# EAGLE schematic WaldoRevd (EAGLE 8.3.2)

## Sheet 1 of 6: Microcontroller Module
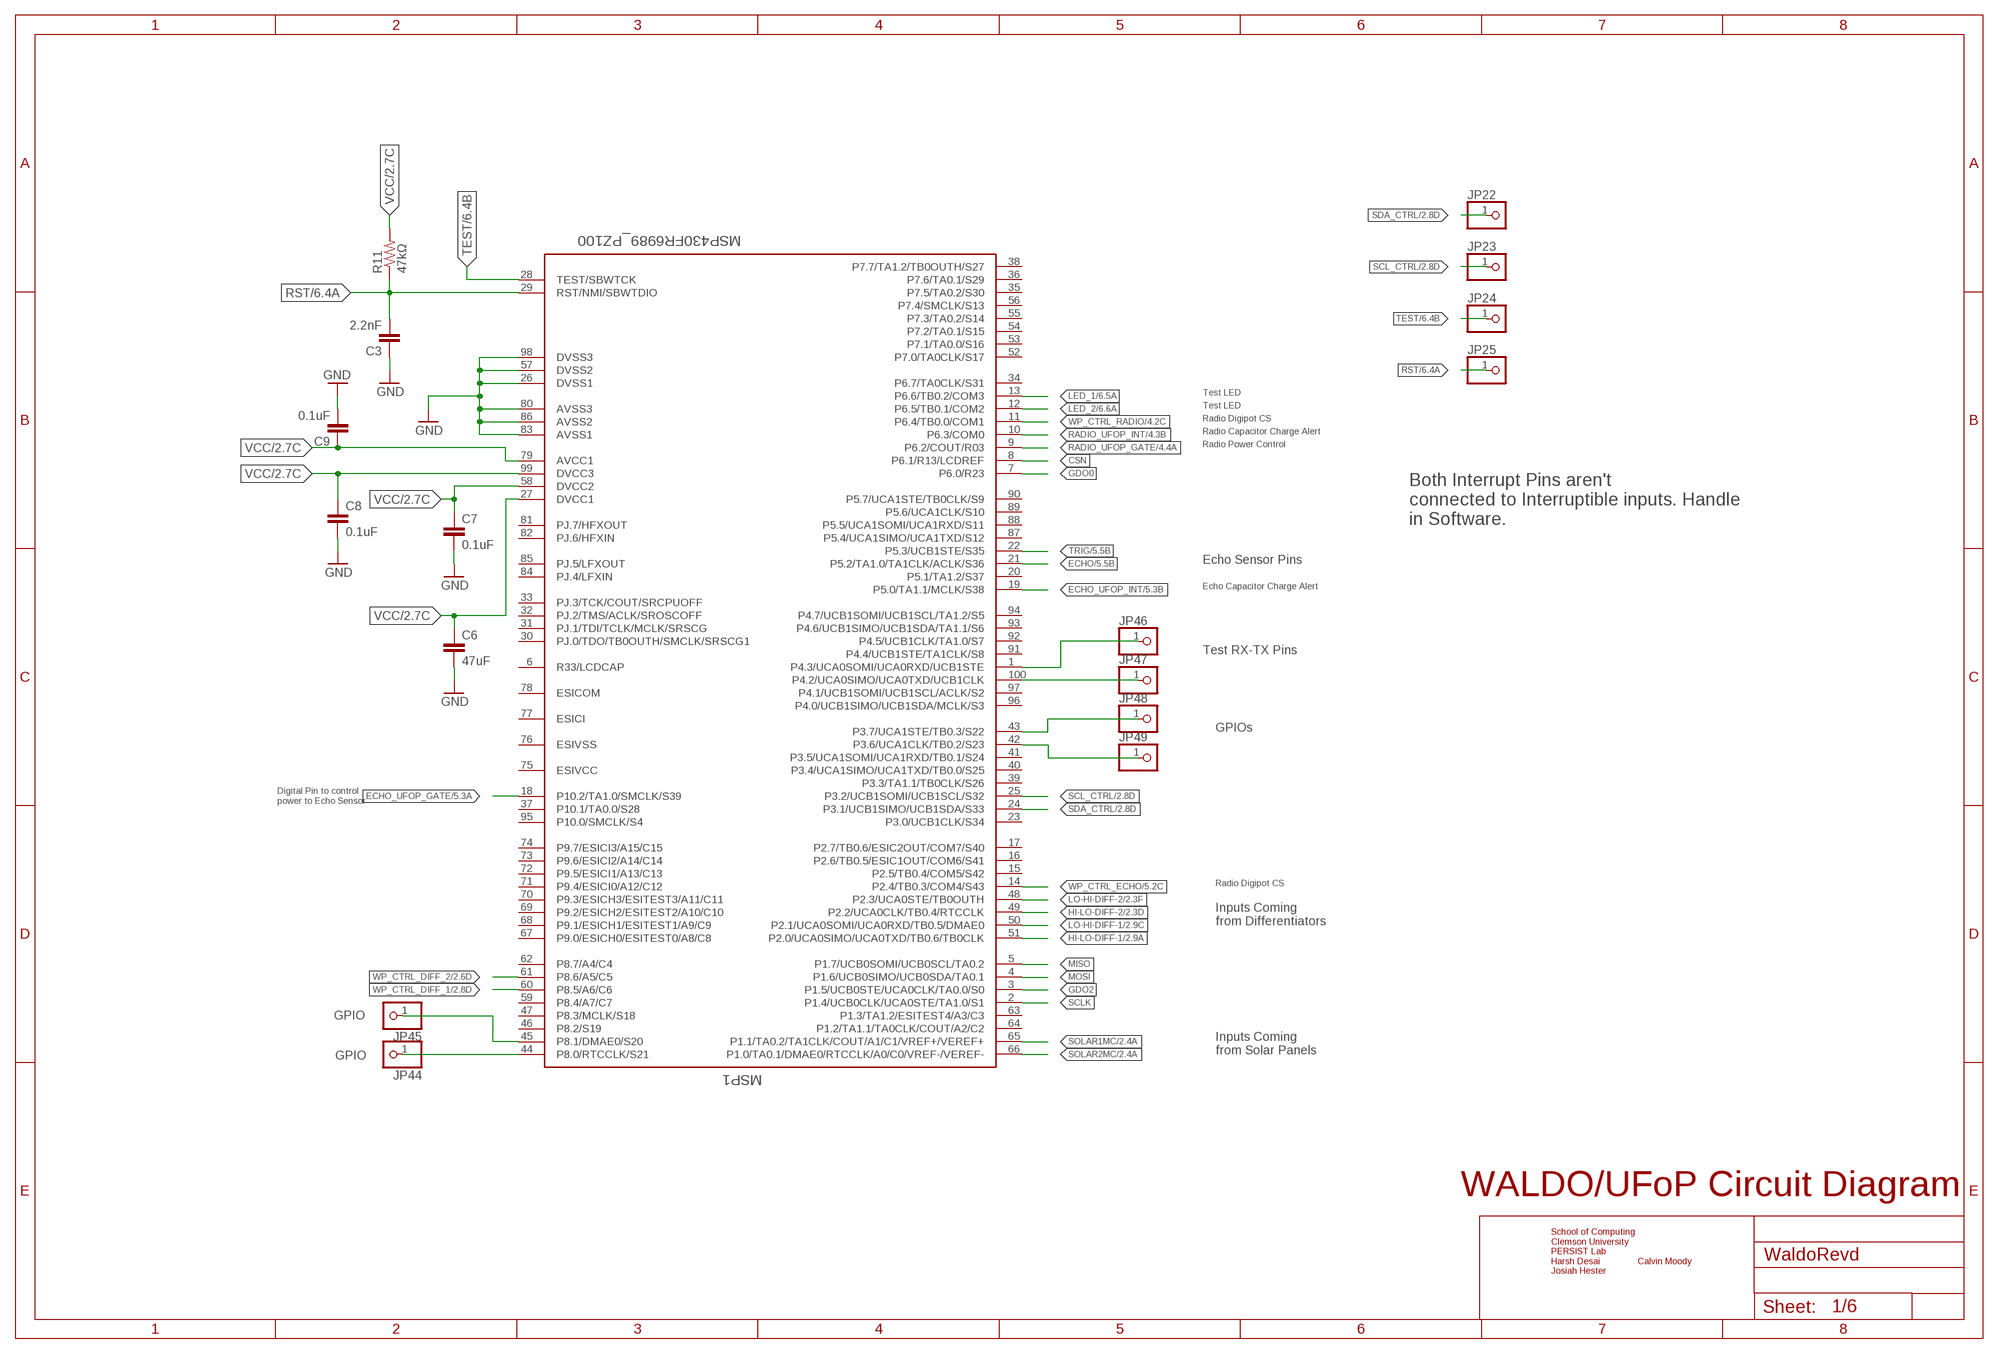
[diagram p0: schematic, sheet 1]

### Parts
C3  2.2nF  CAP0805  [0805]
C6  47uF  CAP0805  [0805]
C7  0.1uF  CAP0805  [0805]
C8  0.1uF  CAP0805  [0805]
C9  0.1uF  CAP0805  [0805]
JP22  PINHD-1X1  [1X01]
JP23  PINHD-1X1  [1X01]
JP24  PINHD-1X1  [1X01]
JP25  PINHD-1X1  [1X01]
JP44  PINHD-1X1  [1X01]
JP45  PINHD-1X1  [1X01]
JP46  PINHD-1X1  [1X01]
JP47  PINHD-1X1  [1X01]
JP48  PINHD-1X1  [1X01]
JP49  PINHD-1X1  [1X01]
MSP1  MSP430FR6989_PZ100  [PZ100]
R11  47kΩ  RESISTOR0805-RES  [0805]

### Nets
CSN: MSP1.8(P6.1/R13/LCDREF) ; also sheet 4
ECHO: MSP1.21(P5.2/TA1.0/TA1CLK/ACLK/S36) ; also sheet 5
ECHO_UFOP_GATE: MSP1.18(P10.2/TA1.0/SMCLK/S39) ; also sheet 5
ECHO_UFOP_INT: MSP1.19(P5.0/TA1.1/MCLK/S38) ; also sheet 5
GDO0: MSP1.7(P6.0/R23) ; also sheet 4
GDO2: MSP1.3(P1.5/UCB0STE/UCA0CLK/TA0.0/S0) ; also sheet 4
GND: C3.1 C6.2 C7.2 C8.2 C9.2 MSP1.26(DVSS1) MSP1.57(DVSS2) MSP1.80(AVSS3) MSP1.83(AVSS1) MSP1.86(AVSS2) MSP1.98(DVSS3) ; also sheet 2,3,4,5,6
HI-LO-DIFF-1: MSP1.51(P2.0/UCA0SIMO/UCA0TXD/TB0.6/TB0CLK) ; also sheet 2
HI-LO-DIFF-2: MSP1.49(P2.2/UCA0CLK/TB0.4/RTCCLK) ; also sheet 2
LED_1: MSP1.13(P6.6/TB0.2/COM3) ; also sheet 6
LED_2: MSP1.12(P6.5/TB0.1/COM2) ; also sheet 6
LO-HI-DIFF-1: MSP1.50(P2.1/UCA0SOMI/UCA0RXD/TB0.5/DMAE0) ; also sheet 2
LO-HI-DIFF-2: MSP1.48(P2.3/UCA0STE/TB0OUTH) ; also sheet 2
MISO: MSP1.5(P1.7/UCB0SOMI/UCB0SCL/TA0.2) ; also sheet 4
MOSI: MSP1.4(P1.6/UCB0SIMO/UCB0SDA/TA0.1) ; also sheet 4
N$1: JP44.1 MSP1.44(P8.0/RTCCLK/S21)
N$2: JP45.1 MSP1.45(P8.1/DMAE0/S20)
N$3: JP46.1 MSP1.1(P4.3/UCA0SOMI/UCA0RXD/UCB1STE)
N$5: JP47.1 MSP1.100(P4.2/UCA0SIMO/UCA0TXD/UCB1CLK)
N$6: JP49.1 MSP1.42(P3.6/UCA1CLK/TB0.2/S23)
N$10: JP48.1 MSP1.43(P3.7/UCA1STE/TB0.3/S22)
RADIO_UFOP_GATE: MSP1.9(P6.2/COUT/R03) ; also sheet 4
RADIO_UFOP_INT: MSP1.10(P6.3/COM0) ; also sheet 4
RST: C3.2 JP25.1 MSP1.29(RST/NMI/SBWTDIO) R11.1 ; also sheet 6
SCL_CTRL: JP23.1 MSP1.25(P3.2/UCB1SOMI/UCB1SCL/S32) ; also sheet 2,4,5,6
SCLK: MSP1.2(P1.4/UCB0CLK/UCA0STE/TA1.0/S1) ; also sheet 4
SDA_CTRL: JP22.1 MSP1.24(P3.1/UCB1SIMO/UCB1SDA/S33) ; also sheet 2,4,5,6
SOLAR1MC: MSP1.65(P1.1/TA0.2/TA1CLK/COUT/A1/C1/VREF+/VEREF+) ; also sheet 2
SOLAR2MC: MSP1.66(P1.0/TA0.1/DMAE0/RTCCLK/A0/C0/VREF-/VEREF-) ; also sheet 2
TEST: JP24.1 MSP1.28(TEST/SBWTCK) ; also sheet 6
TRIG: MSP1.22(P5.3/UCB1STE/S35) ; also sheet 5
VCC: C6.1 C7.1 C8.1 C9.1 MSP1.27(DVCC1) MSP1.58(DVCC2) MSP1.79(AVCC1) MSP1.99(DVCC3) R11.2 ; also sheet 2,3,6
WP_CTRL_DIFF_1: MSP1.60(P8.5/A6/C6) ; also sheet 2
WP_CTRL_DIFF_2: MSP1.61(P8.6/A5/C5) ; also sheet 2
WP_CTRL_ECHO: MSP1.14(P2.4/TB0.3/COM4/S43) ; also sheet 5
WP_CTRL_RADIO: MSP1.11(P6.4/TB0.0/COM1) ; also sheet 4
Unconnected: MSP1.6(R33/LCDCAP) MSP1.15(P2.5/TB0.4/COM5/S42) MSP1.16(P2.6/TB0.5/ESIC1OUT/COM6/S41) MSP1.17(P2.7/TB0.6/ESIC2OUT/COM7/S40) MSP1.20(P5.1/TA1.2/S37) MSP1.23(P3.0/UCB1CLK/S34) MSP1.30(PJ.0/TDO/TB0OUTH/SMCLK/SRSCG1) MSP1.31(PJ.1/TDI/TCLK/MCLK/SRSCG) MSP1.32(PJ.2/TMS/ACLK/SROSCOFF) MSP1.33(PJ.3/TCK/COUT/SRCPUOFF) MSP1.34(P6.7/TA0CLK/S31) MSP1.35(P7.5/TA0.2/S30) MSP1.36(P7.6/TA0.1/S29) MSP1.37(P10.1/TA0.0/S28) MSP1.38(P7.7/TA1.2/TB0OUTH/S27) MSP1.39(P3.3/TA1.1/TB0CLK/S26) MSP1.40(P3.4/UCA1SIMO/UCA1TXD/TB0.0/S25) MSP1.41(P3.5/UCA1SOMI/UCA1RXD/TB0.1/S24) MSP1.46(P8.2/S19) MSP1.47(P8.3/MCLK/S18) MSP1.52(P7.0/TA0CLK/S17) MSP1.53(P7.1/TA0.0/S16) MSP1.54(P7.2/TA0.1/S15) MSP1.55(P7.3/TA0.2/S14) MSP1.56(P7.4/SMCLK/S13) MSP1.59(P8.4/A7/C7) MSP1.62(P8.7/A4/C4) MSP1.63(P1.3/TA1.2/ESITEST4/A3/C3) MSP1.64(P1.2/TA1.1/TA0CLK/COUT/A2/C2) MSP1.67(P9.0/ESICH0/ESITEST0/A8/C8) MSP1.68(P9.1/ESICH1/ESITEST1/A9/C9) MSP1.69(P9.2/ESICH2/ESITEST2/A10/C10) MSP1.70(P9.3/ESICH3/ESITEST3/A11/C11) MSP1.71(P9.4/ESICI0/A12/C12) MSP1.72(P9.5/ESICI1/A13/C13) MSP1.73(P9.6/ESICI2/A14/C14) MSP1.74(P9.7/ESICI3/A15/C15) MSP1.75(ESIVCC) MSP1.76(ESIVSS) MSP1.77(ESICI) MSP1.78(ESICOM) MSP1.81(PJ.7/HFXOUT) MSP1.82(PJ.6/HFXIN) MSP1.84(PJ.4/LFXIN) MSP1.85(PJ.5/LFXOUT) MSP1.87(P5.4/UCA1SIMO/UCA1TXD/S12) MSP1.88(P5.5/UCA1SOMI/UCA1RXD/S11) MSP1.89(P5.6/UCA1CLK/S10) MSP1.90(P5.7/UCA1STE/TB0CLK/S9) MSP1.91(P4.4/UCB1STE/TA1CLK/S8) MSP1.92(P4.5/UCB1CLK/TA1.0/S7) MSP1.93(P4.6/UCB1SIMO/UCB1SDA/TA1.1/S6) MSP1.94(P4.7/UCB1SOMI/UCB1SCL/TA1.2/S5) MSP1.95(P10.0/SMCLK/S4) MSP1.96(P4.0/UCB1SIMO/UCB1SDA/MCLK/S3) MSP1.97(P4.1/UCB1SOMI/UCB1SCL/ACLK/S2)

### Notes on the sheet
- Test LED
- Test LED
- Radio Digipot CS
- Radio Capacitor Charge Alert
- Radio Power Control
- Both Interrupt Pins aren't 
  connected to Interruptible inputs. Handle
  in Software.
- Echo Sensor Pins
- Echo Capacitor Charge Alert
- Test RX-TX Pins
- GPIOs
- Digital Pin to control 
  power to Echo Sensor
- Radio Digipot CS
- Inputs Coming 
  from Differentiators
- GPIO
- Inputs Coming 
  from Solar Panels
- GPIO
- WALDO/UFoP Circuit Diagram
- School of Computing
  Clemson University
  PERSIST Lab
  Harsh Desai               Calvin Moody
  Josiah Hester

## Sheet 2 of 6: Solar Panels + Processing (Differentiators)
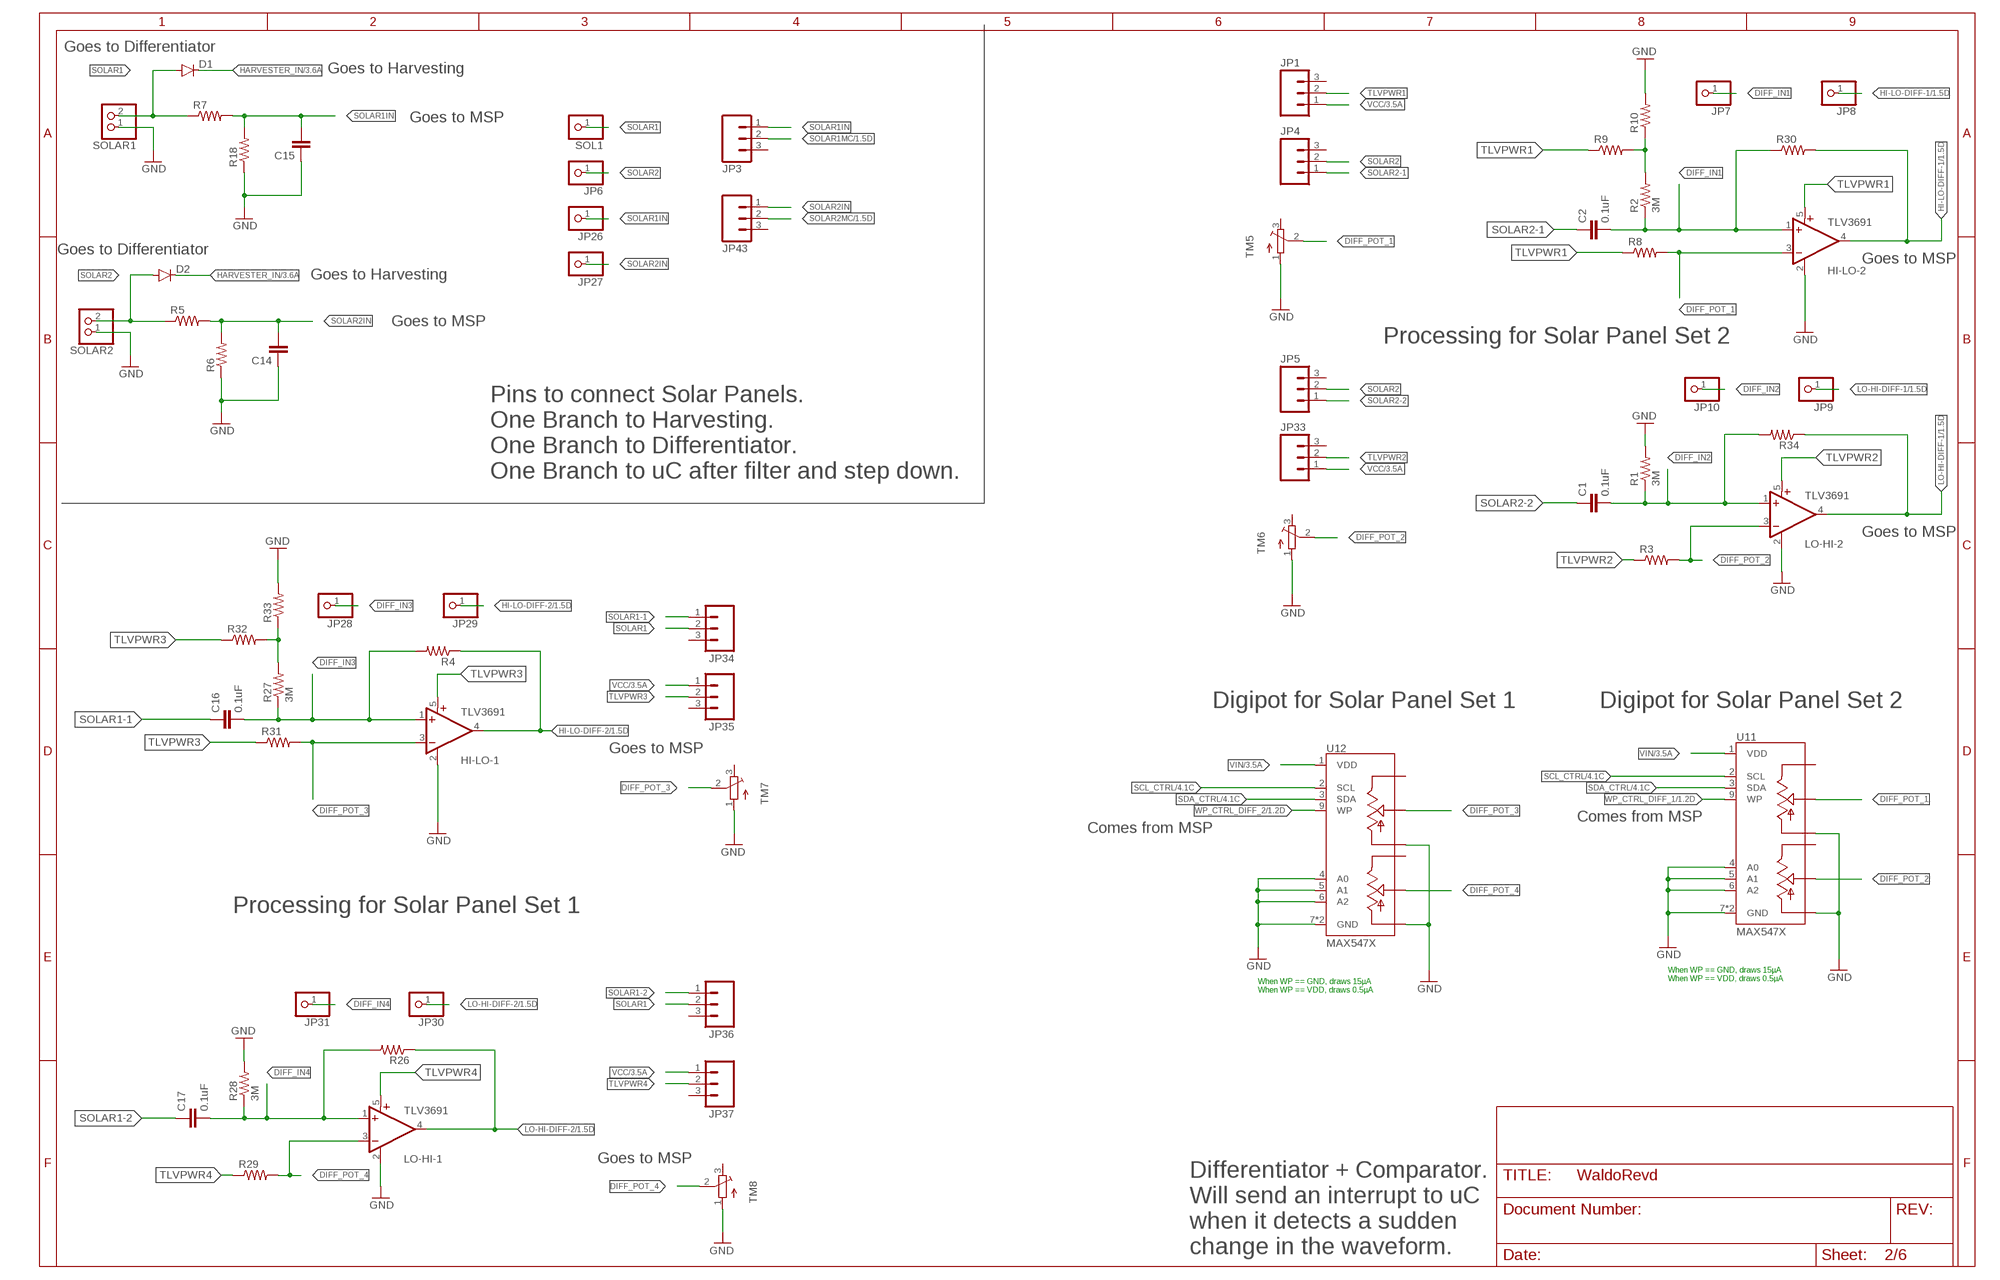
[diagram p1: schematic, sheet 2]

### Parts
C1  0.1uF  CAP0805  [0805]
C2  0.1uF  CAP0805  [0805]
C14  CAP0805  [0805]
C15  CAP0805  [0805]
C16  0.1uF  CAP0805  [0805]
C17  0.1uF  CAP0805  [0805]
D1  DIODESOD523  [SOD523]
D2  DIODESOD523  [SOD523]
HI-LO-1  TLV3691  [SC70-5]
HI-LO-2  TLV3691  [SC70-5]
JP1  M03  [1X03-1.27MM]
JP3  M03  [1X03-1.27MM]
JP4  M03  [1X03-1.27MM]
JP5  M03  [1X03-1.27MM]
JP6  PINHD-1X1  [1X01]
JP7  PINHD-1X1  [1X01]
JP8  PINHD-1X1  [1X01]
JP9  PINHD-1X1  [1X01]
JP10  PINHD-1X1  [1X01]
JP26  PINHD-1X1  [1X01]
JP27  PINHD-1X1  [1X01]
JP28  PINHD-1X1  [1X01]
JP29  PINHD-1X1  [1X01]
JP30  PINHD-1X1  [1X01]
JP31  PINHD-1X1  [1X01]
JP33  M03  [1X03-1.27MM]
JP34  M03  [1X03-1.27MM]
JP35  M03  [1X03-1.27MM]
JP36  M03  [1X03-1.27MM]
JP37  M03  [1X03-1.27MM]
JP43  M03  [1X03-1.27MM]
LO-HI-1  TLV3691  [SC70-5]
LO-HI-2  TLV3691  [SC70-5]
R1  3M  RESISTOR0805-RES  [0805]
R2  3M  RESISTOR0805-RES  [0805]
R3  RESISTOR0805-RES  [0805]
R4  RESISTOR0805-RES  [0805]
R5  RESISTOR0805-RES  [0805]
R6  RESISTOR0805-RES  [0805]
R7  RESISTOR0805-RES  [0805]
R8  RESISTOR0805-RES  [0805]
R9  RESISTOR0805-RES  [0805]
R10  RESISTOR0805-RES  [0805]
R18  RESISTOR0805-RES  [0805]
R26  RESISTOR0805-RES  [0805]
R27  3M  RESISTOR0805-RES  [0805]
R28  3M  RESISTOR0805-RES  [0805]
R29  RESISTOR0805-RES  [0805]
R30  RESISTOR0805-RES  [0805]
R31  RESISTOR0805-RES  [0805]
R32  RESISTOR0805-RES  [0805]
R33  RESISTOR0805-RES  [0805]
R34  RESISTOR0805-RES  [0805]
SOL1  PINHD-1X1  [1X01]
SOLAR1  PINHD-1X2  [1X02]
SOLAR2  PINHD-1X2  [1X02]
TM5  TRIMPOTTC33X  [TC33X]
TM6  TRIMPOTTC33X  [TC33X]
TM7  TRIMPOTTC33X  [TC33X]
TM8  TRIMPOTTC33X  [TC33X]
U11  MAX547X  [QFN16]
U12  MAX547X  [QFN16]

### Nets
DIFF_IN1: C2.2 HI-LO-2.1(+IN) JP7.1 R2.1 R30.1
DIFF_IN2: C1.2 JP10.1 LO-HI-2.1(+IN) R1.1 R34.2
DIFF_IN3: C16.2 HI-LO-1.1(+IN) JP28.1 R4.2 R27.1
DIFF_IN4: C17.2 JP31.1 LO-HI-1.1(+IN) R26.2 R28.1
DIFF_POT_1: HI-LO-2.3(-IN) R8.2 TM5.2(S) U11.14(WA)
DIFF_POT_2: LO-HI-2.3(-IN) R3.2 TM6.2(S) U11.11(WB)
DIFF_POT_3: HI-LO-1.3(-IN) R31.2 TM7.2(S) U12.14(WA)
DIFF_POT_4: LO-HI-1.3(-IN) R29.2 TM8.2(S) U12.11(WB)
GND: C14.1 C15.1 HI-LO-1.2(GND) HI-LO-2.2(GND) LO-HI-1.2(GND) LO-HI-2.2(GND) R1.2 R6.1 R10.2 R18.1 R28.2 R33.2 SOLAR1.1 SOLAR2.1 TM5.1(A) TM6.1(A) TM7.1(A) TM8.1(A) U11.4(A0) U11.5(A1) U11.6(A2) U11.7(GND) U11.10(LB) U11.13(LA) U11.TH(GND) U12.4(A0) U12.5(A1) U12.6(A2) U12.7(GND) U12.10(LB) U12.13(LA) U12.TH(GND) ; also sheet 1,3,4,5,6
HARVESTER_IN: D1.C D2.C ; also sheet 3
HI-LO-DIFF-1: HI-LO-2.4(OUT) JP8.1 R30.2 ; also sheet 1
HI-LO-DIFF-2: HI-LO-1.4(OUT) JP29.1 R4.1 ; also sheet 1
LO-HI-DIFF-1: JP9.1 LO-HI-2.4(OUT) R34.1 ; also sheet 1
LO-HI-DIFF-2: JP30.1 LO-HI-1.4(OUT) R26.1 ; also sheet 1
N$4: R27.2 R32.2 R33.1
N$8: R2.2 R9.2 R10.1
SCL_CTRL: U11.2(SCL) U12.2(SCL) ; also sheet 1,4,5,6
SDA_CTRL: U11.3(SDA) U12.3(SDA) ; also sheet 1,4,5,6
SOLAR1: D1.A JP34.2 JP36.2 R7.1 SOL1.1 SOLAR1.2
SOLAR1-1: C16.1 JP34.1
SOLAR1-2: C17.1 JP36.1
SOLAR1IN: C15.2 JP3.1 JP26.1 R7.2 R18.2
SOLAR1MC: JP3.2 ; also sheet 1
SOLAR2: D2.A JP4.2 JP5.2 JP6.1 R5.1 SOLAR2.2
SOLAR2-1: C2.1 JP4.1
SOLAR2-2: C1.1 JP5.1
SOLAR2IN: C14.2 JP27.1 JP43.1 R5.2 R6.2
SOLAR2MC: JP43.2 ; also sheet 1
TLVPWR1: HI-LO-2.5(V+) JP1.2 R8.1 R9.1
TLVPWR2: JP33.2 LO-HI-2.5(V+) R3.1
TLVPWR3: HI-LO-1.5(V+) JP35.2 R31.1 R32.1
TLVPWR4: JP37.2 LO-HI-1.5(V+) R29.1
VCC: JP1.1 JP33.1 JP35.1 JP37.1 ; also sheet 1,3,6
VIN: U11.1(VDD) U12.1(VDD) ; also sheet 3,4,5,6
WP_CTRL_DIFF_1: U11.9(WP) ; also sheet 1
WP_CTRL_DIFF_2: U12.9(WP) ; also sheet 1
Unconnected: JP1.3 JP3.3 JP4.3 JP5.3 JP33.3 JP34.3 JP35.3 JP36.3 JP37.3 JP43.3 TM5.3(E) TM6.3(E) TM7.3(E) TM8.3(E) U11.12(HB) U11.15(HA) U12.12(HB) U12.15(HA)

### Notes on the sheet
- Goes to Differentiator
- Goes to Harvesting
- Goes to MSP
- Goes to Differentiator
- Goes to MSP
- Goes to Harvesting
- Goes to MSP
- Processing for Solar Panel Set 2
- Pins to connect Solar Panels.
  One Branch to Harvesting.
  One Branch to Differentiator.
  One Branch to uC after filter and step down.
- Goes to MSP
- Digipot for Solar Panel Set 1 | Digipot for Solar Panel Set 2
- Goes to MSP
- Comes from MSP
- Comes from MSP
- Processing for Solar Panel Set 1
- When WP == GND, draws 15µA
  When WP == VDD, draws 0.5µA
- When WP == GND, draws 15µA
  When WP == VDD, draws 0.5µA
- Goes to MSP
- Differentiator + Comparator.
  Will send an interrupt to uC 
  when it detects a sudden 
  change in the waveform.

## Sheet 3 of 6: Battery + Regulator
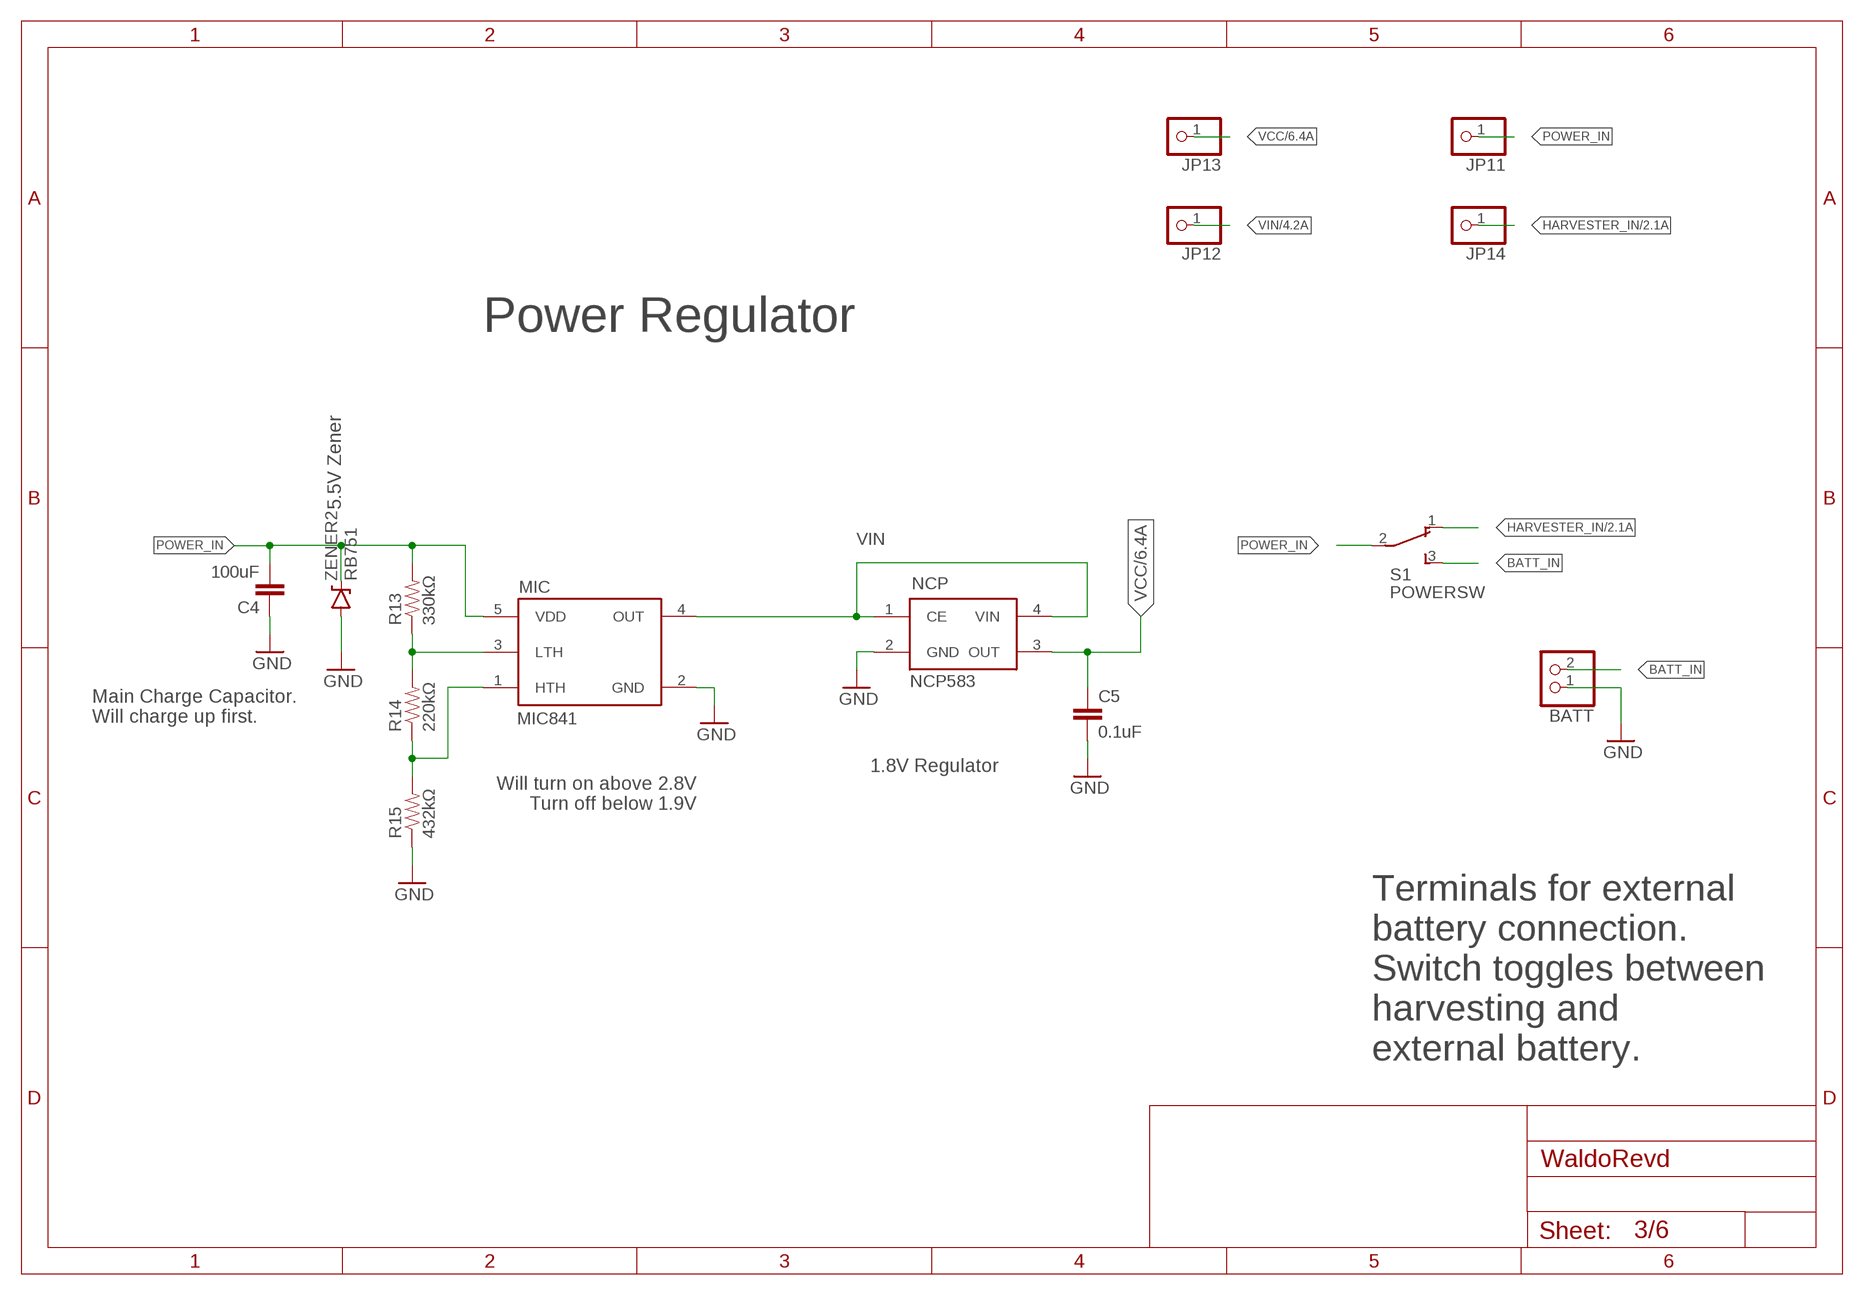
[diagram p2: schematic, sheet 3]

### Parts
BATT  PINHD-1X2  [1X02]
C4  100uF  CAP0805  [0805]
C5  0.1uF  CAP0805  [0805]
JP11  PINHD-1X1  [1X01]
JP12  PINHD-1X1  [1X01]
JP13  PINHD-1X1  [1X01]
JP14  PINHD-1X1  [1X01]
MIC  MIC841  [SC70-5]
NCP  NCP583  [SC82-AB_1PRIMARY]
R13  330kΩ  RESISTOR0805-RES  [0805]
R14  220kΩ  RESISTOR0805-RES  [0805]
R15  432kΩ  RESISTOR0805-RES  [0805]
S1  POWERSW  [TL3XYO]
ZENER2  RB751  DIODE-ZENER  [SOD-523]

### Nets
BATT_IN: BATT.2 S1.3(S)
GND: BATT.1 C4.1 C5.2 MIC.2(GND) NCP.2(GND) R15.1 ZENER2.ANODE(A) ; also sheet 1,2,4,5,6
HARVESTER_IN: JP14.1 S1.1(O) ; also sheet 2
N$11: MIC.3(LTH) R13.1 R14.2
N$12: MIC.1(HTH) R14.1 R15.2
POWER_IN: C4.2 JP11.1 MIC.5(VDD) R13.2 S1.2(P) ZENER2.CATHODE(C)
VCC: C5.1 JP13.1 NCP.3(OUT) ; also sheet 1,2,6
VIN: JP12.1 MIC.4(OUT) NCP.1(CE) NCP.4(VIN) ; also sheet 2,4,5,6

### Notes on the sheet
- Power Regulator
- 5.5V Zener
- Main Charge Capacitor.
  Will charge up first.
- 1.8V Regulator
- Will turn on above 2.8V
  Turn off below 1.9V
- Terminals for external
  battery connection.
  Switch toggles between
  harvesting and 
  external battery.

## Sheet 4 of 6: Radio Module
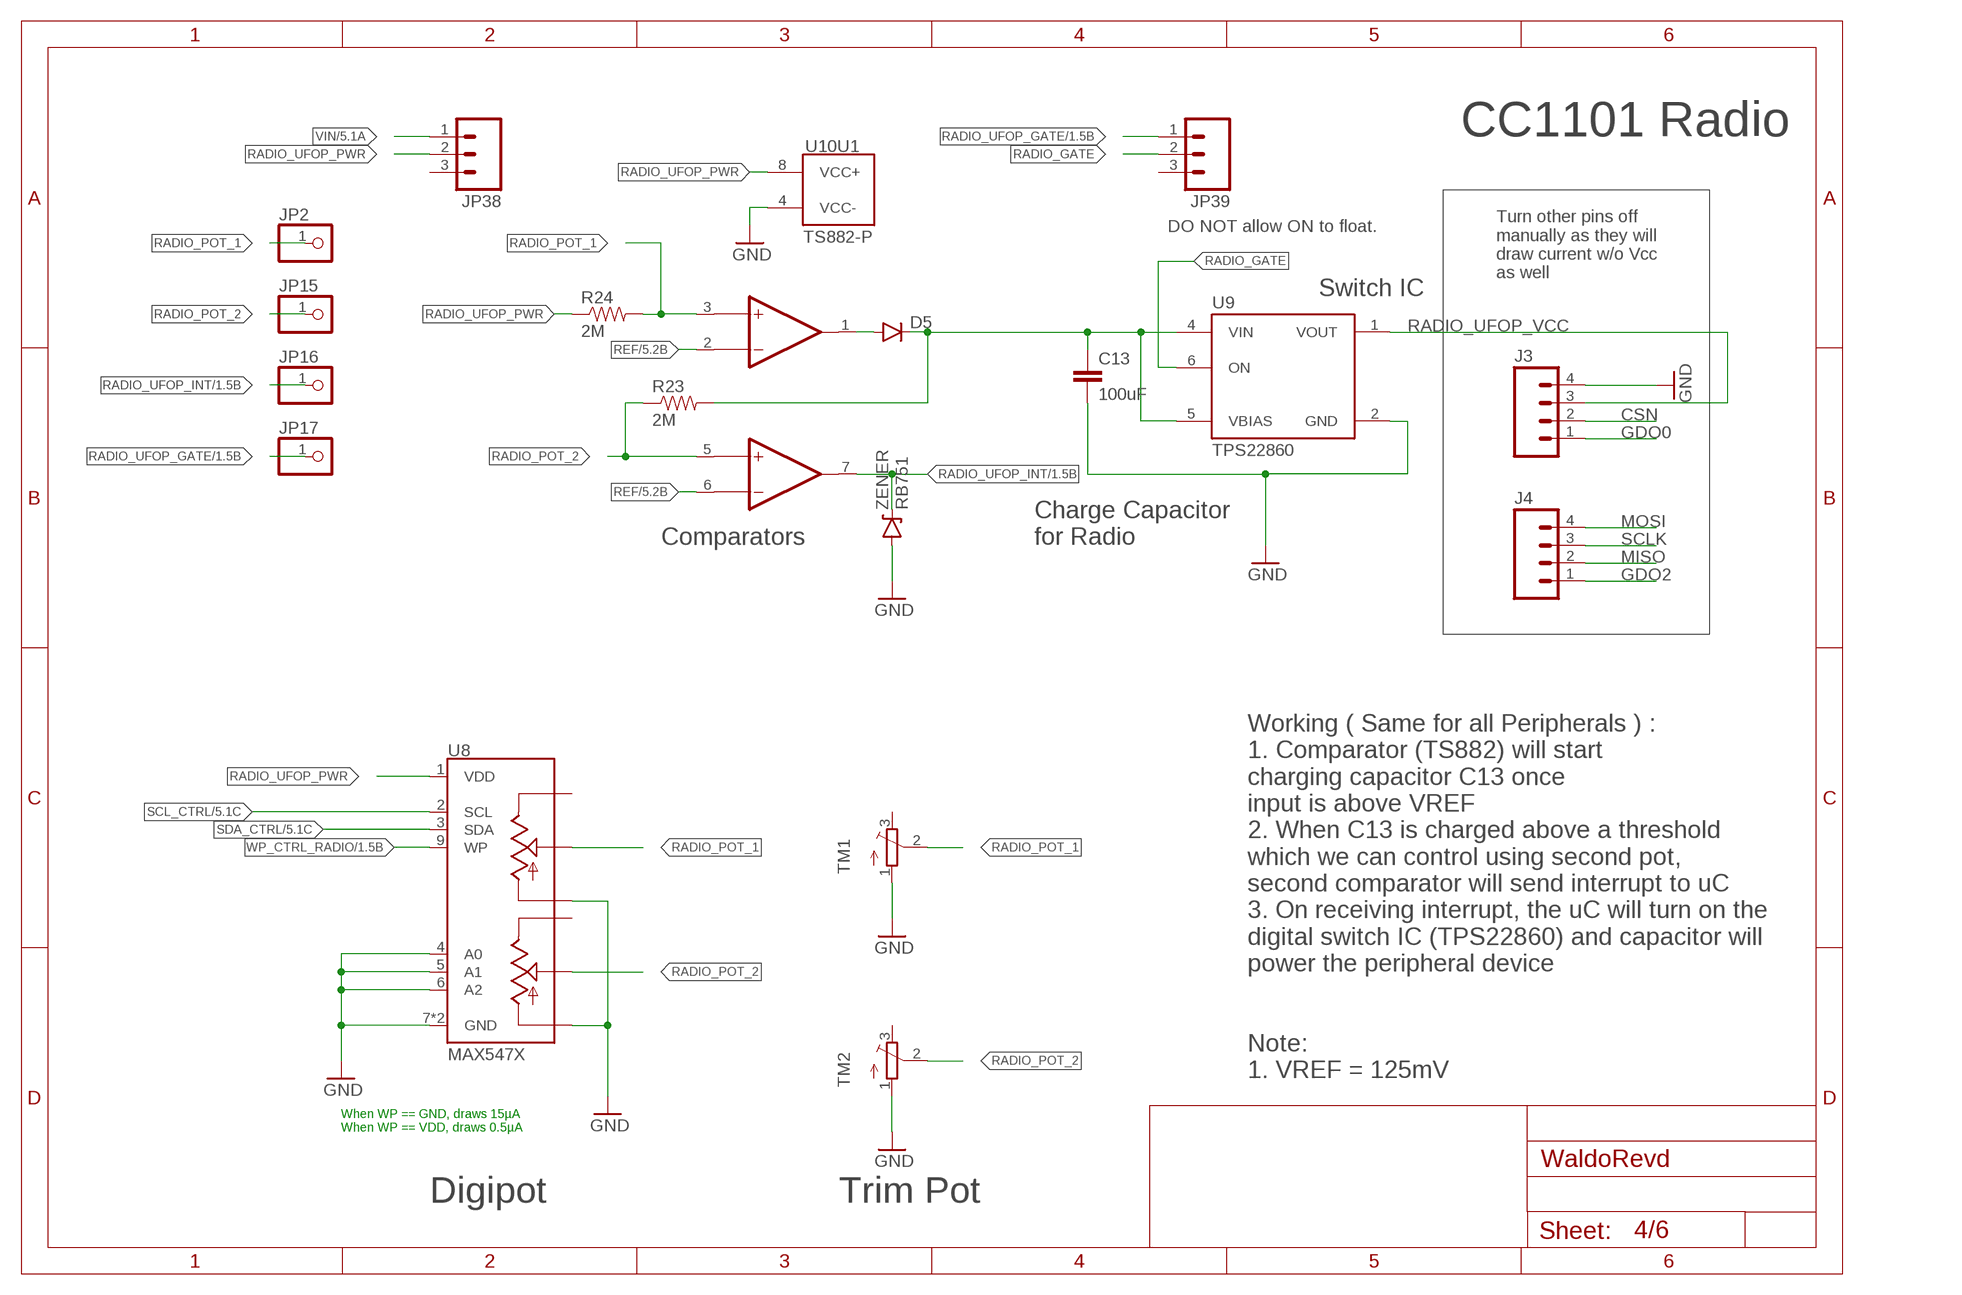
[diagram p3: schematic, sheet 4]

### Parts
C13  100uF  CAP0805  [0805]
D5  DIODESOD523  [SOD523]
J3  M04PTH  [1X04]
J4  M04PTH  [1X04]
JP2  PINHD-1X1  [1X01]
JP15  PINHD-1X1  [1X01]
JP16  PINHD-1X1  [1X01]
JP17  PINHD-1X1  [1X01]
JP38  M03  [1X03-1.27MM]
JP39  M03  [1X03-1.27MM]
R23  2M  RESISTOR0805-RES  [0805]
R24  2M  RESISTOR0805-RES  [0805]
TM1  TRIMPOTTC33X  [TC33X]
TM2  TRIMPOTTC33X  [TC33X]
U8  MAX547X  [QFN16]
U9  TPS22860  [TSOT23-6]
U10  TS882-P  [UDFN8]
ZENER  RB751  DIODE-ZENER  [SOD-523]

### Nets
CSN: J3.2 ; also sheet 1
GDO0: J3.1 ; also sheet 1
GDO2: J4.1 ; also sheet 1
GND: C13.2 J3.4 TM1.1(A) TM2.1(A) U8.4(A0) U8.5(A1) U8.6(A2) U8.7(GND) U8.10(LB) U8.13(LA) U8.TH(GND) U9.2(GND) U10.4(U1:VCC-) ZENER.ANODE(A) ; also sheet 1,2,3,5,6
MISO: J4.2 ; also sheet 1
MOSI: J4.4 ; also sheet 1
N$22: C13.1 D5.C R23.2 U9.4(VIN) U9.5(VBIAS)
N$24: D5.A U10.1(OP1:OUT1)
RADIO_GATE: JP39.2 U9.6(ON)
RADIO_POT_1: JP2.1 R24.2 TM1.2(S) U8.14(WA) U10.3(OP1:IN1+)
RADIO_POT_2: JP15.1 R23.1 TM2.2(S) U8.11(WB) U10.5(OP2:IN1+)
RADIO_UFOP_GATE: JP17.1 JP39.1 ; also sheet 1
RADIO_UFOP_INT: JP16.1 U10.7(OP2:OUT1) ZENER.CATHODE(C) ; also sheet 1
RADIO_UFOP_PWR: JP38.2 R24.1 U8.1(VDD) U10.8(U1:VCC+)
RADIO_UFOP_VCC: J3.3 U9.1(VOUT)
REF: U10.2(OP1:IN1-) U10.6(OP2:IN1-) ; also sheet 5,6
SCL_CTRL: U8.2(SCL) ; also sheet 1,2,5,6
SCLK: J4.3 ; also sheet 1
SDA_CTRL: U8.3(SDA) ; also sheet 1,2,5,6
VIN: JP38.1 ; also sheet 2,3,5,6
WP_CTRL_RADIO: U8.9(WP) ; also sheet 1
Unconnected: JP38.3 JP39.3 TM1.3(E) TM2.3(E) U8.12(HB) U8.15(HA)

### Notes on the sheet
- CC1101 Radio
- DO NOT allow ON to float.
- Turn other pins off 
  manually as they will
  draw current w/o Vcc
  as well
- Switch IC
- Comparators
- Charge Capacitor 
  for Radio
- Working ( Same for all Peripherals ) :
  1. Comparator (TS882) will start 
  charging capacitor C13 once 
  input is above VREF
  2. When C13 is charged above a threshold
  which we can control using second pot, 
  second comparator will send interrupt to uC
  3. On receiving interrupt, the uC will turn on the
  digital switch IC (TPS22860) and capacitor will 
  power the peripheral device
- Note:
  1. VREF = 125mV
- When WP == GND, draws 15µA
  When WP == VDD, draws 0.5µA
- Digipot | Trim Pot

## Sheet 5 of 6: Echo Sensor Module
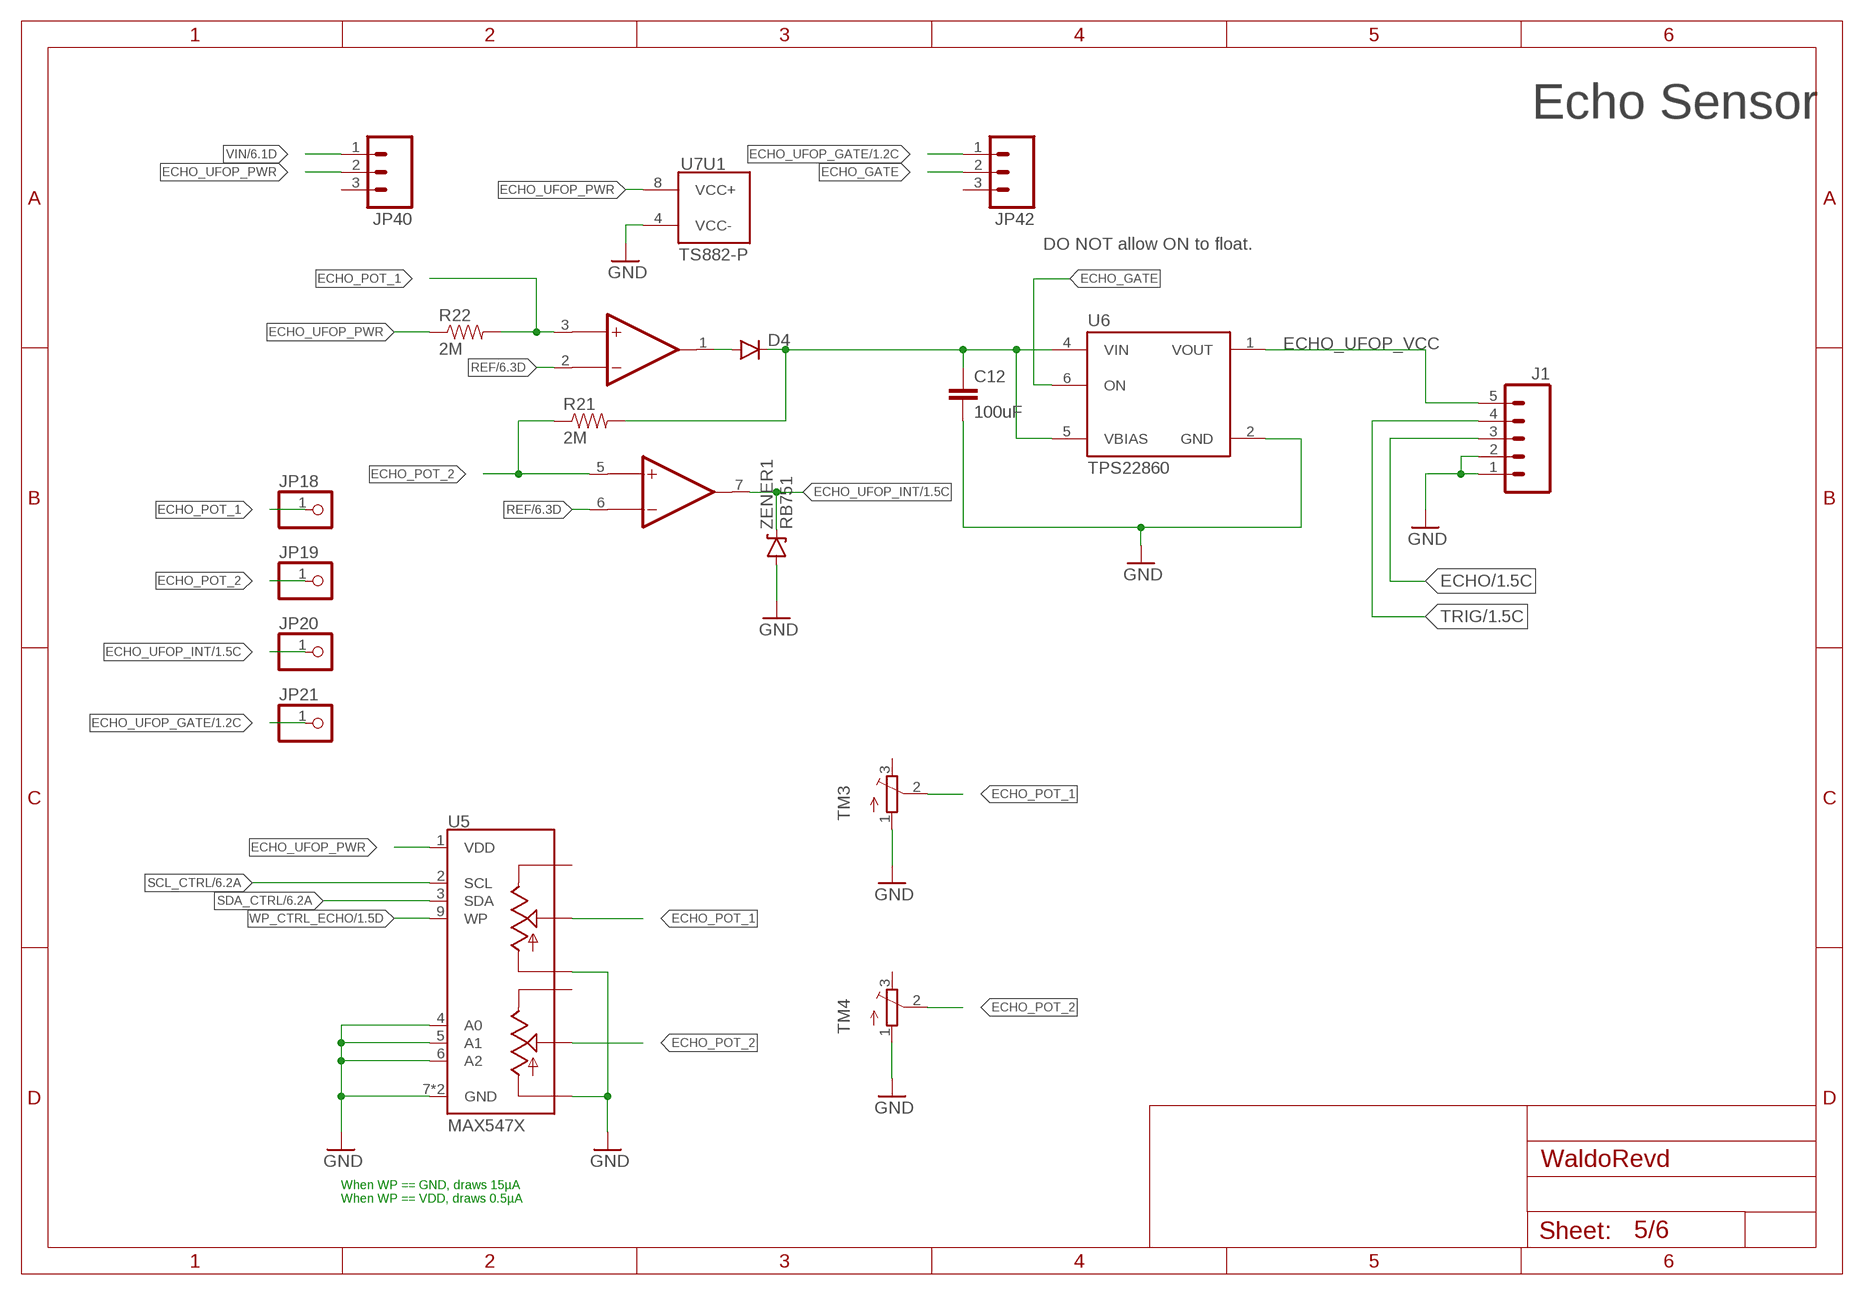
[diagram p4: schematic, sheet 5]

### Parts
C12  100uF  CAP0805  [0805]
D4  DIODESOD523  [SOD523]
J1  M05PTH  [1X05]
JP18  PINHD-1X1  [1X01]
JP19  PINHD-1X1  [1X01]
JP20  PINHD-1X1  [1X01]
JP21  PINHD-1X1  [1X01]
JP40  M03  [1X03-1.27MM]
JP42  M03  [1X03-1.27MM]
R21  2M  RESISTOR0805-RES  [0805]
R22  2M  RESISTOR0805-RES  [0805]
TM3  TRIMPOTTC33X  [TC33X]
TM4  TRIMPOTTC33X  [TC33X]
U5  MAX547X  [QFN16]
U6  TPS22860  [TSOT23-6]
U7  TS882-P  [UDFN8]
ZENER1  RB751  DIODE-ZENER  [SOD-523]

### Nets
ECHO: J1.3 ; also sheet 1
ECHO_GATE: JP42.2 U6.6(ON)
ECHO_POT_1: JP18.1 R22.2 TM3.2(S) U5.14(WA) U7.3(OP1:IN1+)
ECHO_POT_2: JP19.1 R21.1 TM4.2(S) U5.11(WB) U7.5(OP2:IN1+)
ECHO_UFOP_GATE: JP21.1 JP42.1 ; also sheet 1
ECHO_UFOP_INT: JP20.1 U7.7(OP2:OUT1) ZENER1.CATHODE(C) ; also sheet 1
ECHO_UFOP_PWR: JP40.2 R22.1 U5.1(VDD) U7.8(U1:VCC+)
ECHO_UFOP_VCC: J1.5 U6.1(VOUT)
GND: C12.2 J1.1 J1.2 TM3.1(A) TM4.1(A) U5.4(A0) U5.5(A1) U5.6(A2) U5.7(GND) U5.10(LB) U5.13(LA) U5.TH(GND) U6.2(GND) U7.4(U1:VCC-) ZENER1.ANODE(A) ; also sheet 1,2,3,4,6
N$17: C12.1 D4.C R21.2 U6.4(VIN) U6.5(VBIAS)
N$20: D4.A U7.1(OP1:OUT1)
REF: U7.2(OP1:IN1-) U7.6(OP2:IN1-) ; also sheet 4,6
SCL_CTRL: U5.2(SCL) ; also sheet 1,2,4,6
SDA_CTRL: U5.3(SDA) ; also sheet 1,2,4,6
TRIG: J1.4 ; also sheet 1
VIN: JP40.1 ; also sheet 2,3,4,6
WP_CTRL_ECHO: U5.9(WP) ; also sheet 1
Unconnected: JP40.3 JP42.3 TM3.3(E) TM4.3(E) U5.12(HB) U5.15(HA)

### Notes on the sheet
- Echo Sensor
- DO NOT allow ON to float.
- When WP == GND, draws 15µA
  When WP == VDD, draws 0.5µA

## Sheet 6 of 6: Programmer, RTC, Misc
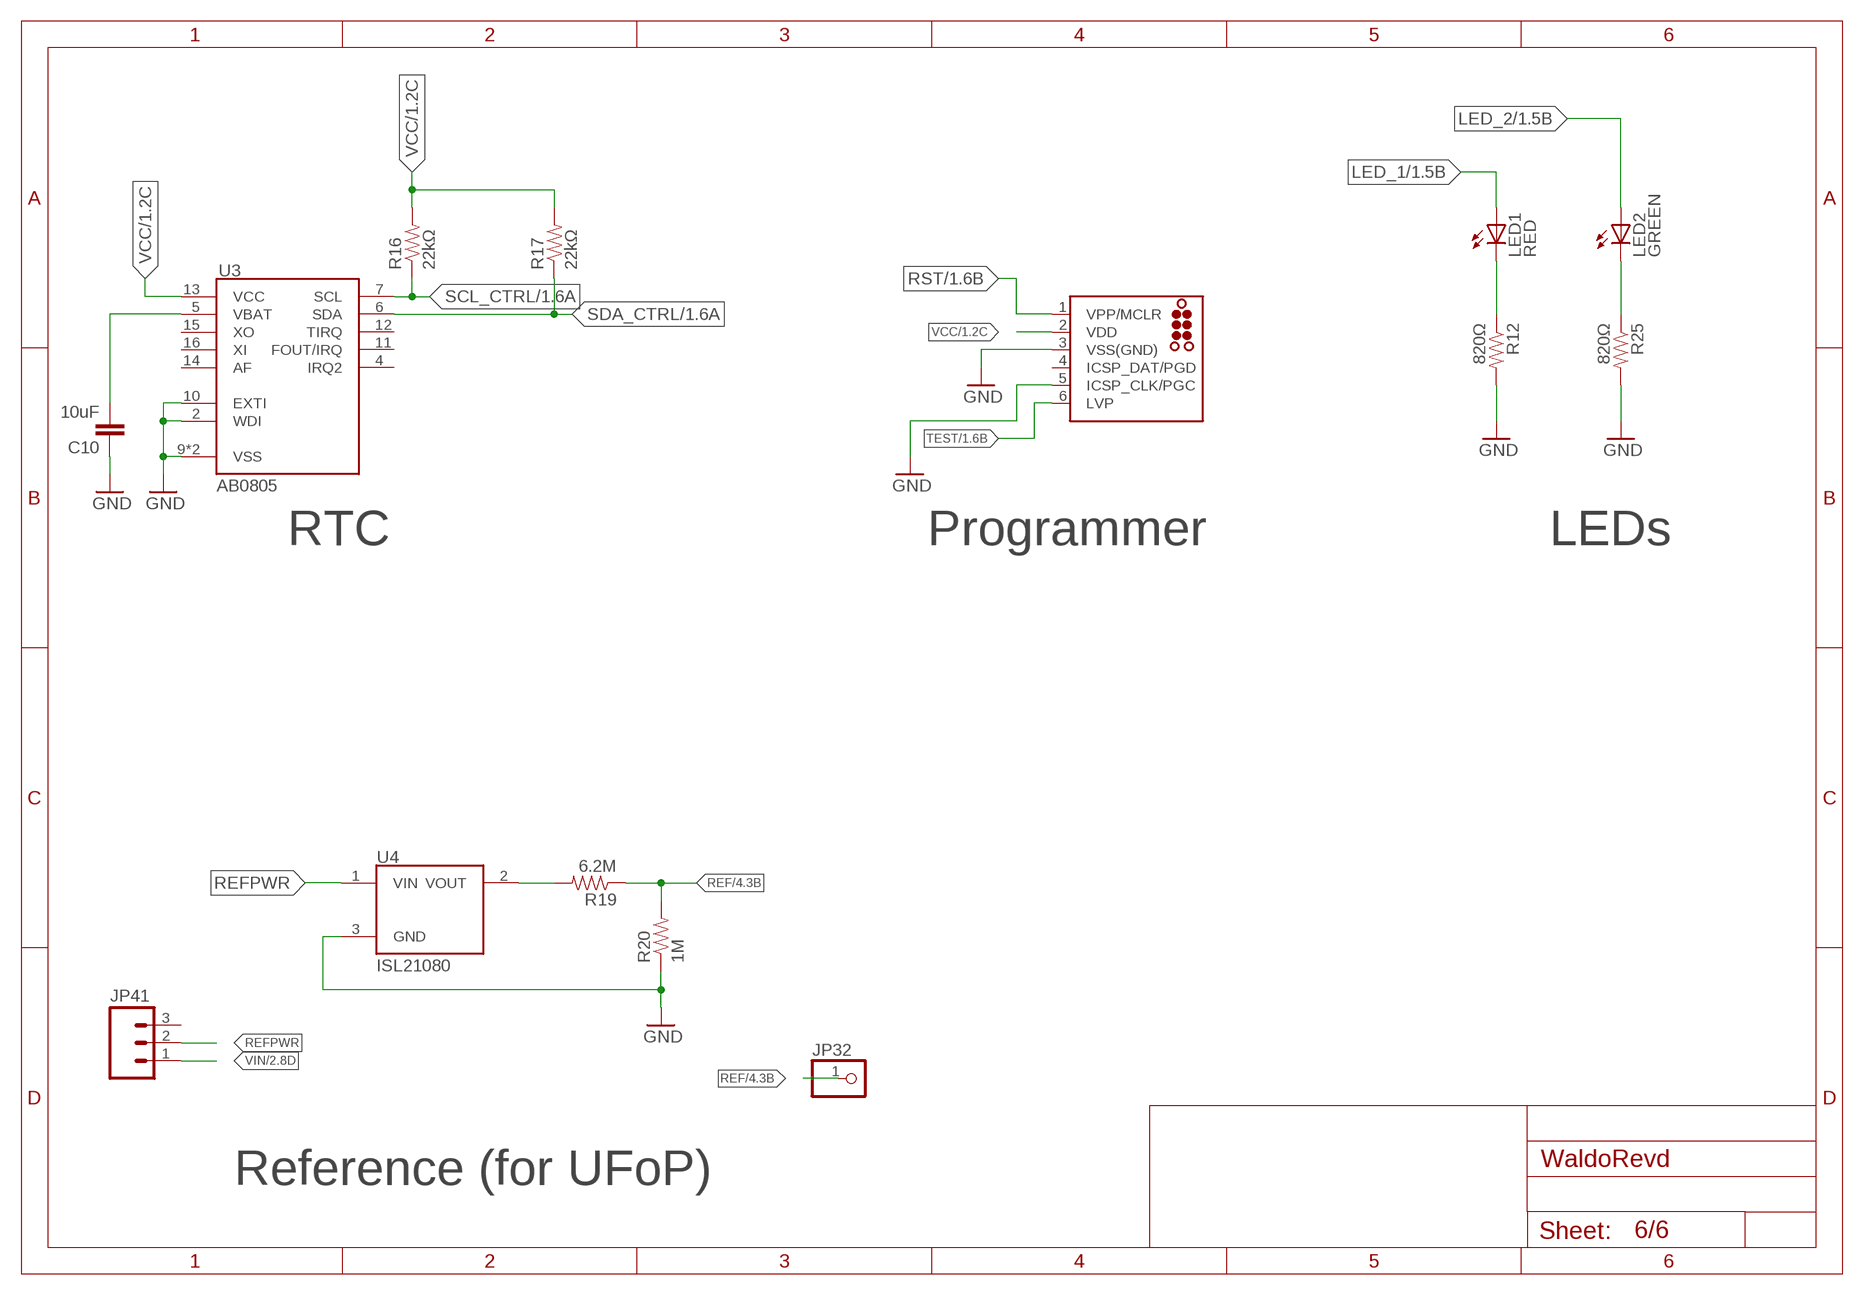
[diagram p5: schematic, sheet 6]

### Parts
C10  10uF  CAP0805  [0805]
J2  TC2030-MCP-NL  [TC2030-MCP-NL]
JP32  PINHD-1X1  [1X01]
JP41  M03  [1X03-1.27MM]
LED1  RED  LEDCHIP-LED0805  [CHIP-LED0805]
LED2  GREEN  LEDCHIP-LED0805  [CHIP-LED0805]
R12  820Ω  RESISTOR0805-RES  [0805]
R16  22kΩ  RESISTOR0805-RES  [0805]
R17  22kΩ  RESISTOR0805-RES  [0805]
R19  6.2M  RESISTOR0805-RES  [0805]
R20  1M  RESISTOR0805-RES  [0805]
R25  820Ω  RESISTOR0805-RES  [0805]
U3  AB0805  [QFN16]
U4  ISL21080  [SOT-23]

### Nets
GND: C10.1 J2.3(VSS(GND)) J2.5(ICSP_CLK/PGC) R12.2 R20.1 R25.2 U3.2(WDI) U3.9(VSS) U3.10(EXTI) U3.TH(VSS) U4.3(GND) ; also sheet 1,2,3,4,5
LED_1: LED1.A ; also sheet 1
LED_2: LED2.A ; also sheet 1
N$7: LED1.C R12.1
N$9: LED2.C R25.1
N$13: C10.2 U3.5(VBAT)
N$14: R19.2 U4.2(VOUT)
REF: JP32.1 R19.1 R20.2 ; also sheet 4,5
REFPWR: JP41.2 U4.1(VIN)
RST: J2.1(VPP/MCLR) ; also sheet 1
SCL_CTRL: R16.1 U3.7(SCL) ; also sheet 1,2,4,5
SDA_CTRL: R17.1 U3.6(SDA) ; also sheet 1,2,4,5
TEST: J2.6(LVP) ; also sheet 1
VCC: J2.2(VDD) R16.2 R17.2 U3.13(VCC) ; also sheet 1,2,3
VIN: JP41.1 ; also sheet 2,3,4,5
Unconnected: J2.4(ICSP_DAT/PGD) JP41.3 U3.4(IRQ2) U3.11(FOUT/IRQ) U3.12(TIRQ) U3.14(AF) U3.15(XO) U3.16(XI)

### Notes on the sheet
- RTC | Programmer | LEDs
- Reference (for UFoP)

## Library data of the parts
BATT SOLAR1 SOLAR2 = pinhead:PINHD-1X2: PIN HEADER
C1-C10 C14-C17 = SparkFun-Capacitors:CAP: Capacitor
C12 C13 = SparkFun-Capacitors:CAP: Capacitor; DIGIKEY: 490-9969-1-ND
D1 D2 D4 D5 = SparkFun-DiscreteSemi:DIODE: Diode
HI-LO-1 HI-LO-2 LO-HI-1 LO-HI-2 = fedpower:TLV3691: 0.9-V to 6.5-V, Nanopower Comparator Datasheets Analog Signal Chain Guide TLV3691 Manufacturer Product Page TLV3691IDPFR Specifications Standard Package 1 CategoryIntegrated Circuits (ICs) FamilyLinear - Comparators Series- Packaging Cut Tape (CT) TypeGeneral Purpose Number of Elements1 Output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
J1 = SparkFun-Connectors:M05: Header 5 Standard 5-pin 0.1" header. Use with straight break away headers (SKU : PRT-00116), right angle break away headers (PRT-00553), swiss pins (PRT-00743), machine pins (PRT-00117), and female headers (PRT-00115). Molex polarized connector foot print use with SKU : PRT-08230 with associated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
J2 = tag-connect_msp430:TC2030: TAG-CONNECT ICSP Connector Manufacturer: Tag-Connect Cable for easy In-Circuit Serial Programming. Designed for Microchip ICD2, suitable for many others. Two variants - one "with legs" (for hands-free fit on PCB) and another "without legs" for quick programming. PADDescription 1MCLR/Vpp 2Vdd 3GND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
J3 J4 = SparkFun-Connectors:M04: Header 4 Standard 4-pin 0.1" header. Use with straight break away headers (SKU : PRT-00116), right angle break away headers (PRT-00553), swiss pins (PRT-00743), machine pins (PRT-00117), and female headers (PRT-00115). Molex polarized connector foot print use with SKU : PRT-08231 with associated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; PROD_ID: CONN-09696
JP1 JP3-JP5 JP33-JP43 = SparkFun-Connectors:M03: Header 3 Standard 3-pin 0.1" header. Use with straight break away headers (SKU : PRT-00116), right angle break away headers (PRT-00553), swiss pins (PRT-00743), machine pins (PRT-00117), and female headers (PRT-00115). Molex polarized connector foot print use with SKU : PRT-08232 with associated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
JP2 JP6-JP32 JP44-JP49 SOL1 = adafruit:PINHD-1X1: Pin header 1x1 for 0.1" spacing
LED1 LED2 = led:LED: LED
MIC = mic841:MIC841: MIC841:Comparator with reference and adj. hysteresis
MSP1 = msp430:MSP430FR6989_PZ100
NCP = ncp583:NCP583: NCP583 - Ultra-Low Iq 150 mA CMOS LDO Regulator with Enable The NCP583 series of low dropout regulators are designed for portable battery powered applications which require precise output voltage accuracy and low quiescent current. These devices feature an enable function which lowers current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
R1-R18 R22 R24-R34 = SparkFun-Resistors:RESISTOR: Resistor
R19 = SparkFun-Resistors:RESISTOR: Resistor; DIGIKEY: 541-6.20MHCT-ND
R20 = SparkFun-Resistors:RESISTOR: Resistor; DIGIKEY: 311-1.00MHRCT-ND
R21 R23 = SparkFun-Resistors:RESISTOR: Resistor; DIGIKEY: 311-2.00MHRCT-ND
S1 = GreenBoard:POWERSW: TINY SWITCH ON - ON Source: http://www2.produktinfo.conrad.com/datenblaetter/700000-724999/705152-da-01-de-Subminiaturschalter_TL_36YO.pdf
TM1-TM8 = adafruit:TRIMPOT: SMT trimmer potentiometer part number TC33X http://www.ladyada.net/library/eagle
U3 = AB08XX:AB0805: AB08X5 Real-Time Clock Family: I2C Version The ABRACON AB08X5 Real-Time Clock family provides a groundbreaking combination of ultra-low power coupled with a highly sophisticated feature set. With power requirements significantly lower than any other industry RTC (as low as 14 nA), these are the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; MOUSER: 815-AB0805-T3
U4 = isl21080:ISL21080: Intersil: ISL21080, 300nA NanoPower Voltage References The ISL21080 analog voltage references feature low supply voltage operation at ultra-low 310nA typ, 1.5µA max operating current. Additionally, the ISL21080 family features guaranteed initial accuracy as low as ±0.2% and 50ppm/°C temperature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; DIGIKEY: ISL21080DIH309Z-TKCT-ND
U5 U8 U11 U12 = max547x:MAX547X: MAXIM MAX547X: Dual, 256-Tap, Nonvolatile, I2C-Interface, Digital Potentiometers, 400nA Iq, 250µA 12ms write The MAX5477/MAX5478/MAX5479 nonvolatile, dual, linear-taper, digital potentiometers perform the function of a mechanical potentiometer, but replace the mechanics with a simple 2-wire digital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; DIGIKEY: MAX5479ETE+-ND
U6 U9 = tps22860:TPS22860: TI: TPS22860 Ultra-Low Leakage Load Switch The TPS22860 is a small, ultra-low leakage current, single channel load switch. The device requires a VBIAS voltage and can operate over an input voltage range of 0 V to VBIAS. It can support a maximum continuous current of 200 mA. The switch is controlled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; DIGIKEY: 296-43982-1-ND
U7 U10 = ts882:TS882-P; DIGIKEY: 497-14073-1-ND
ZENER ZENER1 ZENER2 = Parts:DIODE-ZENER: Zener Diode

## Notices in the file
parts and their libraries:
SparkFun-Capacitors: Licensing: Creative Commons ShareAlike 4.0 International - https://creativecommons.org/licenses/by-sa/4.0
tag-connect_msp430: ©2009 ROFA.cz - modified and updated by Robert Darlington ‹rdarlington@gmail.com›
